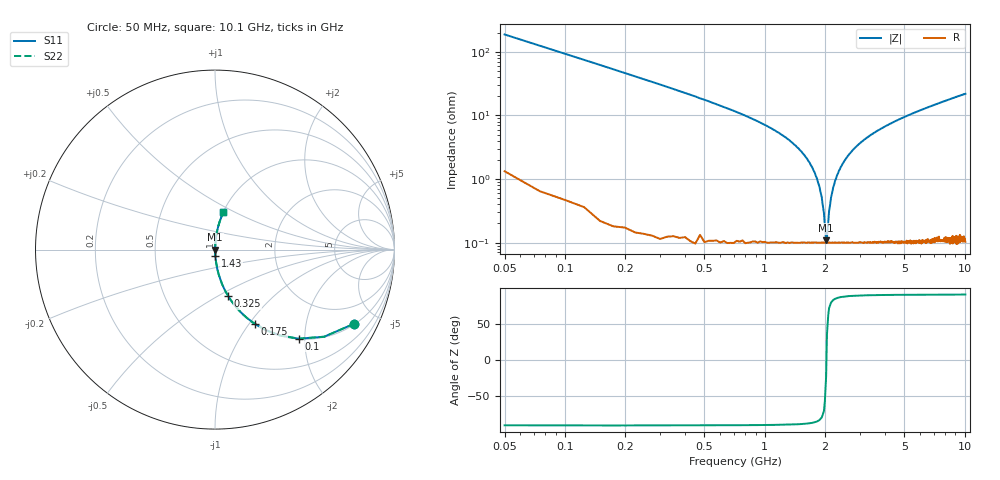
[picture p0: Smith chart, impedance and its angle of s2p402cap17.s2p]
! AVX Thin Film Operation		Date: April 2003
! Description: Accu-P® Series, Thin Film, SMD, RF Capacitor
! Part Number: 04023K170FBS
! 50 MHz  -  10.05 GHz
! Serial Measurements
# hz S db R 50
!	S11		S21		S12		S22
!	dB	Phase	dB	Phase	dB	Phase	dB	Phase
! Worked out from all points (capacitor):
!   400 points, 50 MHz to 10.1 GHz, reference 50 ohm
!   read as one part in series: C = 17 pF near 100 MHz
!   lowest |Z| = 109 mohm at 2.03 GHz (marker M1)
!   series resonance near 2.038 GHz, so ESL is about 360 pH
!   S11 on the Smith chart (normalised r, x): 50 MHz: 1.03, -3.74; 100 MHz: 1.01, -1.87; 175 MHz: 1.00, -1.06; 325 MHz: 1.00, -0.56; 1.43 GHz: 1.00, -0.07; 10.1 GHz: 1.00, +0.44
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5e7  -1.12 -28.0  -6.56 61.6  -6.56 61.6  -1.12 -28.0
1e8  -3.34 -46.8  -2.74 42.9  -2.74 42.9  -3.34 -46.8
1.75e8  -6.59 -61.9  -1.09 27.9  -1.09 27.9  -6.59 -61.9
3.25e8  -11.40 -74.1  -0.34 15.7  -0.34 15.7  -11.40 -74.1
7e8  -18.60 -82.8  -0.07 6.7  -0.07 6.7  -18.60 -82.8
1.43e9  -29.50 -86.4  -0.01 1.9  -0.01 1.9  -29.50 -86.4
1.73e9  -36.30 -85.4  -0.01 0.9  -0.01 0.9  -36.30 -85.4
1.83e9  -40.00 -83.7  -0.01 0.6  -0.01 0.6  -40.00 -83.7
1.93e9  -45.70 -78.6  -0.01 0.3  -0.01 0.3  -45.70 -78.6
1.98e9  -50.70 -69.7  -0.01 0.2  -0.01 0.2  -50.70 -69.7
2.03e9  -59.30 -23.1  -0.01 0.0  -0.01 0.0  -59.30 -23.1
2.05e9  -58.30 35.0  -0.01 -0.0  -0.01 -0.0  -58.30 35.0
2.1e9  -50.20 70.9  -0.01 -0.2  -0.01 -0.2  -50.20 70.9
2.15e9  -45.70 78.6  -0.01 -0.3  -0.01 -0.3  -45.70 78.6
2.25e9  -40.60 83.3  -0.01 -0.5  -0.01 -0.5  -40.60 83.3
2.35e9  -37.50 84.9  -0.01 -0.8  -0.01 -0.8  -37.50 84.9
2.75e9  -31.00 86.3  -0.01 -1.6  -0.01 -1.6  -31.00 86.3
3.4e9  -26.10 86.0  -0.02 -2.8  -0.02 -2.8  -26.10 86.0
5.08e9  -20.40 83.9  -0.05 -5.5  -0.05 -5.5  -20.40 83.9
6.75e9  -17.20 81.7  -0.09 -7.9  -0.09 -7.9  -17.20 81.7
8.43e9  -15.10 79.5  -0.15 -10.2  -0.15 -10.2  -15.10 79.5
1.01e10  -13.40 77.4  -0.21 -12.3  -0.21 -12.3  -13.40 77.4
